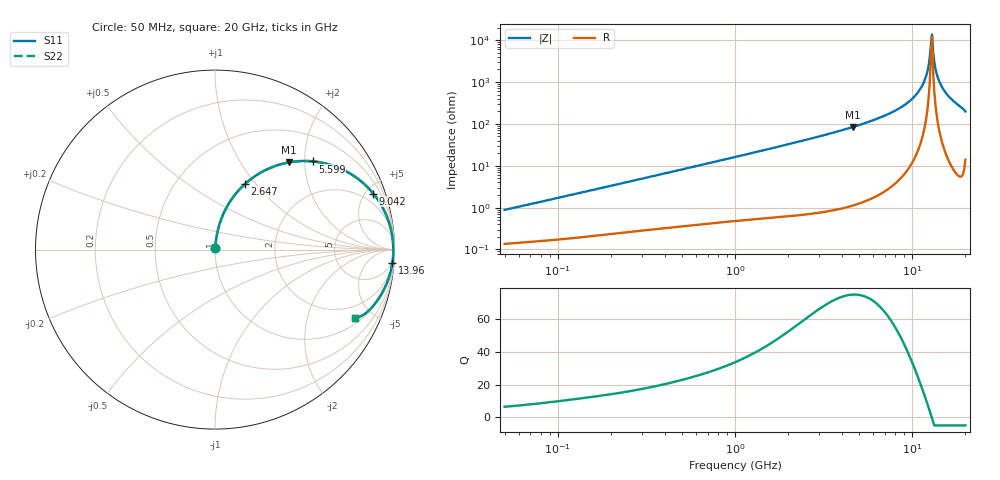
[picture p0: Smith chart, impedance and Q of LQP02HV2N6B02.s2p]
!Murata Part Number: LQP02HV2N6B02
!These Parameters are Measured in Series Mode Connection
!  o--[Z]--o
!Port1  Port2
!  o-------o
!Freq. Start=50[MHz] Stop=20[GHz], 401[Steps]
# Hz S RI R 50
!Freq.(Hz) S11(Real) S11(Imag) S21(Real) S21(Imag) S12(Real) S12(Imag) S22(Real) S22(Imag)
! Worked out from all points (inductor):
!   401 points, 50 MHz to 20 GHz, reference 50 ohm
!   read as one part in series: L = 2.75 nH near 51.52 MHz
!   highest Q = 75.2 at 4.608 GHz (marker M1), where L = 2.89 nH
!   self-resonance near 12.76 GHz
!   S11 on the Smith chart (normalised r, x): 50 MHz: 1.00, +0.02; 2.647 GHz: 1.01, +0.88; 5.599 GHz: 1.03, +2.19; 9.042 GHz: 1.13, +5.62; 13.96 GHz: 3, -26; 20 GHz: 1.28, -3.95
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5e7  0.00143 0.00871  0.9986 -0.00871  0.9986 -0.00871  0.00143 0.00871
1.364002e8  0.00248 0.0228  0.9975 -0.0228  0.9975 -0.0228  0.00248 0.0228
3.721004e8  0.00676 0.0602  0.9932 -0.0602  0.9932 -0.0602  0.00676 0.0602
1e9  0.0298 0.1557  0.9702 -0.1557  0.9702 -0.1557  0.0298 0.1557
2.647493e9  0.1657 0.3639  0.8343 -0.3639  0.8343 -0.3639  0.1657 0.3639
2.728004e9  0.1746 0.3718  0.8254 -0.3718  0.8254 -0.3718  0.1746 0.3718
4.608136e9  0.4136 0.4859  0.5864 -0.4859  0.5864 -0.4859  0.4136 0.4859
5.598765e9  0.5439 0.4913  0.4561 -0.4913  0.4561 -0.4913  0.5439 0.4913
7.442007e9  0.7536 0.4228  0.2464 -0.4228  0.2464 -0.4228  0.7536 0.4228
9.041845e9  0.8821 0.3115  0.1179 -0.3115  0.1179 -0.3115  0.8821 0.3115
1.034674e10  0.948 0.2058  0.052 -0.2058  0.052 -0.2058  0.948 0.2058
1.149051e10  0.9804 0.1116  0.0196 -0.1116  0.0196 -0.1116  0.9804 0.1116
1.201863e10  0.9884 0.0691  0.0116 -0.0691  0.0116 -0.0691  0.9884 0.0691
1.220001e10  0.9902 0.0548  0.00975 -0.0548  0.00975 -0.0548  0.9902 0.0548
1.257102e10  0.9927 0.0259  0.00732 -0.0259  0.00732 -0.0259  0.9927 0.0259
1.276073e10  0.9933 0.0114  0.00674 -0.0114  0.00674 -0.0114  0.9933 0.0114
1.314879e10  0.9931 -0.0176  0.00685 0.0176  0.00685 0.0176  0.9931 -0.0176
1.354865e10  0.9913 -0.0466  0.00867 0.0466  0.00867 0.0466  0.9913 -0.0466
1.396067e10  0.9878 -0.0754  0.0122 0.0754  0.0122 0.0754  0.9878 -0.0754
1.460232e10  0.9794 -0.1182  0.0206 0.1182  0.0206 0.1182  0.9794 -0.1182
1.573793e10  0.9571 -0.1872  0.0429 0.1872  0.0429 0.1872  0.9571 -0.1872
2e10  0.7805 -0.38  0.2195 0.38  0.2195 0.38  0.7805 -0.38
